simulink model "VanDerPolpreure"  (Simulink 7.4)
settings: Solver=ode45  StartTime=0.0  StopTime=100  MaxStep=0.05  RelTol=1e-3
libraries: simulink x1

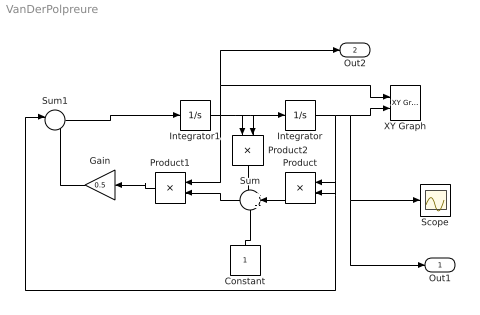
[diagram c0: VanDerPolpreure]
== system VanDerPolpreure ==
  Constant : Constant  OutDataType=sfix(16)  OutScaling=2^0
  Gain : Gain  Gain=0.5  ParameterDataType=sfix(16)  ParameterScaling=2^0  OutDataType=sfix(16)  OutScaling=2^0
  Integrator : Integrator  InitialCondition=0.1
  Integrator1 : Integrator
  Product : Product  OutDataType=sfix(16)  OutScaling=2^0
  Product1 : Product  OutDataType=sfix(16)  OutScaling=2^0
  Product2 : Product  OutDataType=sfix(16)  OutScaling=2^0
  Scope : Scope
  Sum : Sum  Inputs=++-  OutDataType=sfix(16)  OutScaling=2^0
  Sum1 : Sum  Inputs=|--  OutDataType=sfix(16)  OutScaling=2^0
  XY Graph : simulink/Sinks/XY Graph  SystemSampleTime=-1  xmin=-3  xmax=3  ymin=-3  ymax=3  st=-1
  Out1 : Outport  OutDataType=sfix(16)  OutScaling=2^0
  Out2 : Outport  Port=2  OutDataType=sfix(16)  OutScaling=2^0
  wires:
  Integrator/1 -> Product/1, Product/2, Sum1/1, XY Graph/2, Scope/1, Out1/1
  Integrator1/1 -> Product1/1, XY Graph/1, Out2/1, Product2/1, Integrator/1, Product2/2
  Sum/1 -> Product1/2
  Product1/1 -> Gain/1
  Gain/1 -> Sum1/2
  Sum1/1 -> Integrator1/1
  Product2/1 -> Sum/1
  Product/1 -> Sum/2
  Constant/1 -> Sum/3
